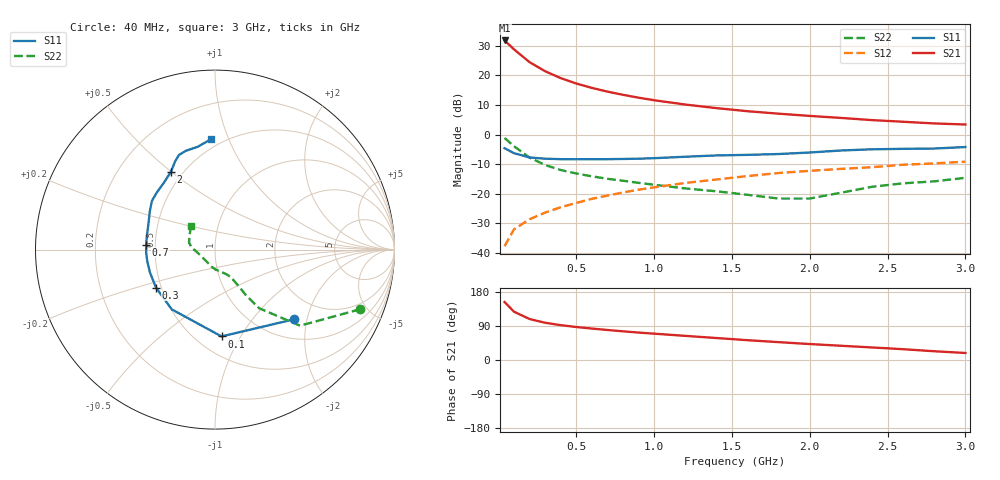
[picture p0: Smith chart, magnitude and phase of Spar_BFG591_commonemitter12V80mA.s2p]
! Filename:  BFG591H.S2P  Version:  4.0
! NXP part #: BFG591  Date: Jun 1994
! Bias condition: Vce=12V; Ic=80mA
#  MHz  S  MA  R  50
! Freq  S11  S21  S12  S22  !GUM [dB]
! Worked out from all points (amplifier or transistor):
!   21 points, 40 MHz to 3 GHz, reference 50 ohm
!   highest |S21| = 31.8 dB at 40 MHz (marker M1)
!   |S21| within 3 dB of that: start of sweep to 100 MHz
!   unconditionally stable (mu >= 1): 614.4 MHz to 2.197 GHz
!   at 300 MHz: K = 0.84, MSG = 23.9 dB, |S12| = -26.4 dB
!   at 1 GHz: K = 1.05, MAG = 13.4 dB, |S12| = -17.9 dB
!   at 3 GHz: K = 0.95, MSG = 6.3 dB, |S12| = -9.2 dB
!   S11 on the Smith chart (normalised r, x): 40 MHz: 1.42, -1.68; 100 MHz: 0.66, -0.83; 300 MHz: 0.47, -0.23; 700 MHz: 0.45, +0.03; 2 GHz: 0.43, +0.50; 3 GHz: 0.44, +0.87
40  0.588 -41.3  38.97 153.0  0.013 72.8  0.875 -22.3
100  0.485 -85.7  27.59 127.5  0.025 62.0  0.636 -41.8
200  0.411 -125.9  16.77 108.2  0.037 60.1  0.409 -53.0
300  0.391 -147.2  11.77 98.3  0.048 62.7  0.306 -55.9
400  0.384 -160.5  9.01 92.0  0.059 64.5  0.252 -56.8
500  0.383 -170.0  7.296 87.1  0.07 66.1  0.22 -57.9
600  0.384 -177.8  6.157 83.0  0.082 66.8  0.197 -58.9
700  0.384 175.8  5.328 79.2  0.093 67.0  0.179 -60.3
800  0.387 169.6  4.703 75.7  0.105 67.0  0.166 -62.1
900  0.391 163.5  4.204 72.4  0.117 67.1  0.153 -64.7
1000  0.399 158.1  3.808 69.5  0.128 66.7  0.142 -68.4
1200  0.422 149.3  3.219 63.7  0.152 65.2  0.123 -77.9
1400  0.444 142.4  2.801 58.0  0.174 63.4  0.11 -89.5
1600  0.454 135.7  2.483 52.3  0.199 62.1  0.096 -102.3
1800  0.469 127.4  2.255 47.1  0.224 59.1  0.083 -120.1
2000  0.498 119.6  2.067 42.1  0.244 57.2  0.083 -149.9
2200  0.538 114.5  1.912 37.6  0.263 55.0  0.104 -174.0
2400  0.564 110.9  1.756 33.1  0.281 54.0  0.131 174.9
2600  0.574 106.3  1.646 28.5  0.309 50.3  0.15 164.7
2800  0.581 99.5  1.543 23.1  0.326 46.3  0.162 151.2
3000  0.616 92.0  1.479 18.5  0.348 44.8  0.186 135.8
